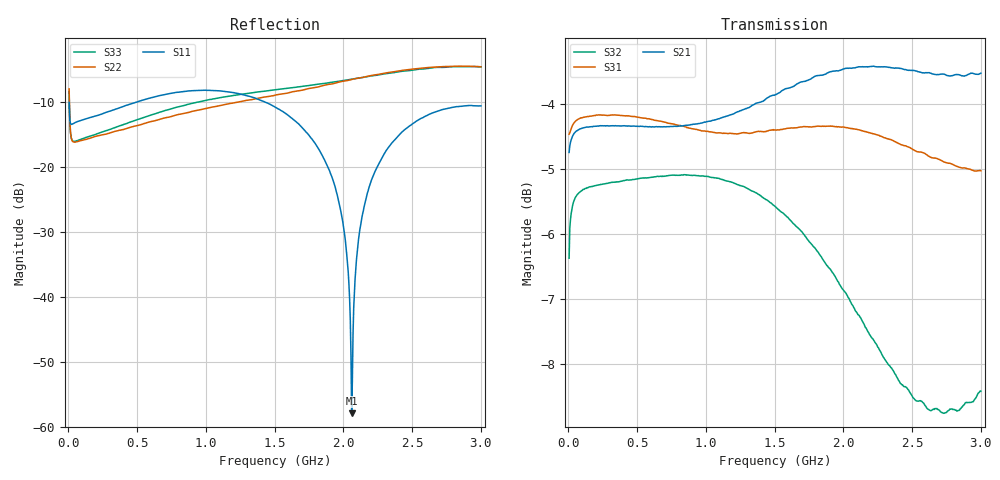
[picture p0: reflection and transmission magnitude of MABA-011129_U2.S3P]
!Agilent Technologies,E5071C,MY46630996,B.13.30
!Date: Tue Aug 16 21:28:03 2022 DD
!Data & Calibration Information:
!MABA-011129-TB soldered onto PT-0028476 with SMA connectors, Port1 (pin1) Port2 (pin4) Port3 (pin3)
!Freq	S11:SOLT3(ON)	S12:SOLT3(ON)	S13:SOLT3(ON)
!	S21:SOLT3(ON)	S22:SOLT3(ON)	S23:SOLT3(ON)
!	S31:SOLT3(ON)	S32:SOLT3(ON)	S33:SOLT3(ON)
!PortZ  Port1:50+j0  Port2:50+j0  Port3:50+j0
!Above PortZ is port z conversion or system Z0 setting when saving the data.
!When reading, reference impedance value at option line is always used.
# Hz S dB R 50
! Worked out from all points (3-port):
!   600 points, 5 MHz to 3 GHz, reference 50 ohm
!   strongest paths, dB at 5 MHz, 755 MHz, 1.505 GHz, 2.255 GHz, 3 GHz:
!     S21: -4.7, -4.4, -3.9, -3.4, -3.5
!     S31: -4.5, -4.3, -4.4, -4.5, -5.0
!     S32: -6.4, -5.1, -5.6, -7.7, -8.4
!   lowest |S11| = -57.9 dB at 2.06 GHz (marker M1), VSWR 1.00, Z = 49.9 + j0.0742 ohm
!   |S11| at or under -10 dB: start of sweep to 497.8 MHz; 1.428 GHz to end of sweep
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5000000  -10.07 61.9  -4.81 -165.7  -4.50 12.3
         -4.75 -165.7  -7.98 94.0  -6.35 31.1
         -4.47 12.3  -6.37 31.1  -8.37 90.9
4.5e7  -13.21 4.6  -4.45 178.4  -4.28 -1.6
       -4.45 178.5  -16.18 24.2  -5.46 2.9
       -4.28 -1.7  -5.47 2.9  -16.06 20.0
6.15e8  -9.28 -99.4  -4.37 126.8  -4.19 -52.6
        -4.36 126.7  -12.96 -53.2  -5.14 -28.7
        -4.25 -52.6  -5.13 -28.8  -11.90 -69.1
1.505e9  -10.80 164.2  -3.90 51.2  -4.40 -128.5
         -3.86 50.8  -8.93 -95.7  -5.60 -76.9
         -4.40 -127.6  -5.58 -77.7  -8.12 -116.1
1.925e9  -22.06 123.8  -3.54 13.5  -4.40 -165.3
         -3.50 12.9  -7.18 -107.9  -6.58 -99.9
         -4.35 -165.0  -6.60 -100.4  -6.94 -127.9
2.015e9  -31.46 115.6  -3.50 5.2  -4.43 -173.5
         -3.46 4.6  -6.74 -110.9  -6.87 -104.3
         -4.37 -173.3  -6.90 -104.8  -6.64 -130.3
2.06e9  -57.89 144.3  -3.49 0.9  -4.43 -177.8
        -3.46 0.4  -6.54 -112.5  -7.10 -106.6
        -4.38 -177.5  -7.07 -107.0  -6.50 -131.6
2.125e9  -29.01 -75.9  -3.48 -4.9  -4.48 176.5
         -3.43 -5.5  -6.26 -114.8  -7.26 -109.5
         -4.41 176.5  -7.28 -109.8  -6.27 -133.5
2.28e9  -18.64 -89.0  -3.47 -19.3  -4.56 162.2
        -3.44 -19.7  -5.64 -121.0  -7.88 -115.9
        -4.51 162.2  -7.85 -116.0  -5.74 -138.4
3e9  -10.59 -139.0  -3.60 -83.1  -5.02 97.1
     -3.53 -82.7  -4.57 -151.2  -8.63 -137.2
     -5.03 96.9  -8.41 -136.9  -4.61 -163.7
